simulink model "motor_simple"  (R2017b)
settings: Solver=VariableStepAuto  StartTime=0.0  StopTime=10.0  RelTol=1e-3
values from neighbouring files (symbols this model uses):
  Ce = 0.33    [init.m]
  Cm = 0.33    [init.m]
  DL = 10    [init.m]
  KL = 100000    [init.m]
  Lm = 0.01    [init.m]
  Rc = 0.4    [init.m]
  Rm = 8.6    [init.m]
undefined symbols (not defined in the file or in its folder): JL, Jm

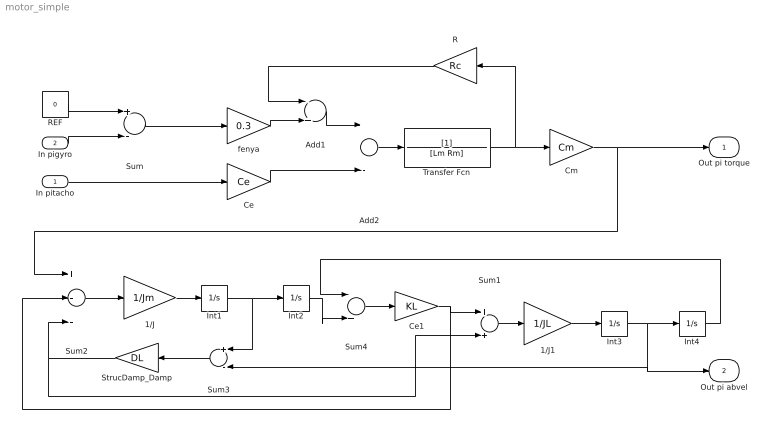
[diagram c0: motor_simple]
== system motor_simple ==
  In pitacho : Inport
  In pigyro : Inport  Port=2
  1/J : Gain  Gain=1/Jm
  1/J1 : Gain  Gain=1/JL
  Add1 : Sum  Inputs=-+
  Add2 : Sum  Inputs=+-
  Ce : Gain  Gain=Ce
  Ce1 : Gain  Gain=KL
  Cm : Gain  Gain=Cm
  Int{1..4} (4 alike) : Integrator
  R : Gain  Gain=Rc
  REF : Constant  Value=0
  StrucDamp_Damp : Gain  Gain=DL
  Sum : Sum  Inputs=+-
  Sum1 : Sum
  Sum2 : Sum  Inputs=+--
  Sum3 : Sum  Inputs=+-
  Sum4 : Sum  Inputs=-+
  Transfer Fcn : TransferFcn  Denominator=[Lm Rm]
  fenya : Gain  Gain=0.3
  Out pi torque : Outport
  Out pi abvel : Outport  Port=2
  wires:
  Cm/1 -> Sum2/1, Out pi torque/1
  In pitacho/1 -> Ce/1
  Transfer Fcn/1 -> R/1, Cm/1
  Ce/1 -> Add2/2
  Add1/1 -> Add2/1
  Add2/1 -> Transfer Fcn/1
  In pigyro/1 -> Sum/2
  REF/1 -> Sum/1
  fenya/1 -> Add1/2
  Sum/1 -> fenya/1
  R/1 -> Add1/1
  Sum4/1 -> Ce1/1
  Sum3/1 -> StrucDamp_Damp/1
  Int2/1 -> Sum4/2
  1/J/1 -> Int1/1
  Sum2/1 -> 1/J/1
  Int4/1 -> Sum4/1
  Ce1/1 -> Sum2/2, Sum1/1
  Int3/1 -> Out pi abvel/1, Sum3/2, Int4/1
  Int1/1 -> Sum3/1, Int2/1
  StrucDamp_Damp/1 -> Sum1/2, Sum2/3
  1/J1/1 -> Int3/1
  Sum1/1 -> 1/J1/1
